(* 	
	Program Name: 	ACS_WRITE_AXIS_BITS
	Purpose:		(To be used only by Output Scan Function) Copy Drive Bits from shadow memory to output registers 
*)
PROGRAM ACS_WRITE_AXIS_BITS
VAR_IN_OUT
	Axis:ACS_DRIVE_TYPE;
END_VAR

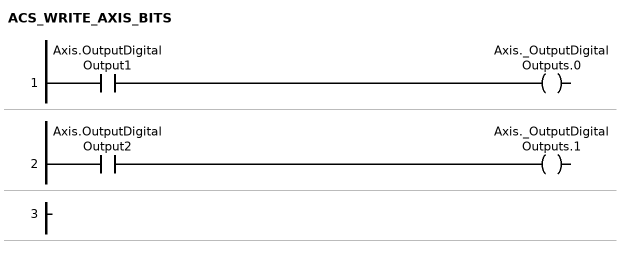
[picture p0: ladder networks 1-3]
// NETWORK 1
Axis._OutputDigitalOutputs.0 := Axis.OutputDigitalOutput1;

// NETWORK 2
Axis._OutputDigitalOutputs.1 := Axis.OutputDigitalOutput2;

// NETWORK 3

END_PROGRAM
